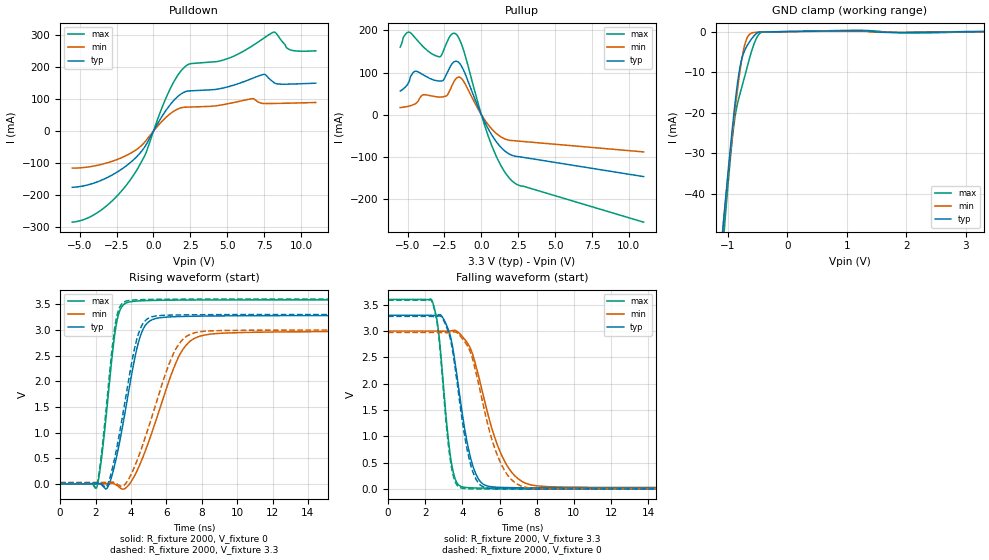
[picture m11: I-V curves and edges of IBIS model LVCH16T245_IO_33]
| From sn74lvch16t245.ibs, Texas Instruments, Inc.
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[Model]   LVCH16T245_IO_33
Model_type  I/O
Vinl=0.8
Vinh=2.0
Enable   Active-Low
Vref =   0
Rref =   2000
Cref =   15p
Vmeas =   1.5
| variable   typ   min   max
C_comp   6.04pF   5.05pF   7.40pF
| C_pullup   14.21pF   6.31pF   25.41pF
| C_pulldown   9.42pF   6.50pF   14.94pF
| C_tri-state   6.04pF   5.05pF   7.40pF
[Temperature Range]   40   100   -40
| Ambient temperature   25   85   -40
[Voltage range]   3.3   3   3.6
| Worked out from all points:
|   slope of the pulldown table from 0 to 0.495 V, typ, clamps not added: 12.4 ohm
|   slope of the pullup table from 0 to 0.495 V, typ, clamps not added: 14 ohm
|   GND clamp passes 1 mA (typ) near -0.56 V on its own axis
|   rising waveform, R_fixture 2000, V_fixture 0: 20-80 % time 1.06ns typ, 1.81ns min, 655ps max; typ from 0 V to 3.28 V
|   falling waveform, R_fixture 2000, V_fixture 3.3: 20-80 % time 887ps typ, 1.47ns min, 565ps max; typ from 3.3 V to 0.019 V
|   rising waveform, R_fixture 2000, V_fixture 3.3: 20-80 % time 1.03ns typ, 1.71ns min, 639ps max; typ from 0.019 V to 3.3 V
|   falling waveform, R_fixture 2000, V_fixture 0: 20-80 % time 841ps typ, 1.32ns min, 547ps max; typ from 3.28 V to 0 V
[GND Clamp]
| LVCH16T245_IO_33
|   Voltage   I(typ)   I(min)   I(max)
-5.5V     -898.4mA   -832.8mA   -1.017A
-1.095V   -50.42mA   -50.2mA    -55.28mA
-1.065V   -45.5mA    -45.64mA   -49.74mA
-1.04V    -41.45mA   -41.9mA    -45.21mA
-970mV    -30.49mA   -31.69mA   -33.19mA
-905mV    -21.04mA   -22.72mA   -23.79mA
-815mV    -10.36mA   -11.66mA   -16.39mA
-725mV    -4.895mA   -3.736mA   -11.48mA
-625mV    -2.267mA   -545.8uA   -5.994mA
-515mV    -439uA     -162.2uA   -1.527mA
-420mV    -95.51uA   -88.06uA   -143.5uA
3.3V      35.84pA    398.7nA    -4.252uA
[Pulldown]
| LVCH16T245_IO_33
|   Voltage   I(typ)   I(min)   I(max)
-5.5V     -176.2mA   -116.1mA   -285.6mA
-3.565V   -154.8mA   -104.8mA   -248.3mA
-1.62V    -100.7mA   -71.19mA   -156.1mA
-535mV    -45.52mA   -31.12mA   -71.38mA
1.155V    84.06mA    55.16mA    134.7mA
2.23V     124.7mA    75.07mA    205.2mA
5.1V      139.6mA    86.34mA    228.5mA
6.75V     166.1mA    101.8mA    268.8mA
7.495V    178.1mA    86.65mA    292mA
8.17V     152.3mA    86.77mA    310.5mA
9.2V      147.4mA    87.68mA    256mA
11V       150.3mA    89.74mA    251.8mA
[Pullup]
| LVCH16T245_IO_33
|   Voltage   I(typ)   I(min)   I(max)
-5.5V     56.18mA    16.98mA    160.3mA
-4.89V    79.66mA    20.64mA    195.7mA
-4.445V   103.3mA    26.89mA    180.5mA
-3.945V   94.62mA    47.4mA     161.1mA
-2.805V   79.84mA    41.85mA    137.4mA
-2.095V   114.9mA    61.02mA    187.6mA
-1.66V    126.5mA    87.57mA    189.1mA
-1.24V    108mA      81.18mA    156.3mA
695mV     -47.39mA   -33.41mA   -72.26mA
1.475V    -82.35mA   -55.39mA   -129.6mA
2.255V    -98mA      -61.58mA   -161.7mA
11V       -146.5mA   -88.02mA   -254.5mA
[Ramp]
| LVCH16T245_IO_33
| variable   typ   min   max
dV/dt_r   2.03/1.10E-09   1.85/1.88E-09   2.20/6.72E-10
dV/dt_f   1.97/8.89E-10   1.79/1.47E-09   2.16/5.70E-10
R_load = 2000
[Rising Waveform]
| LVCH16T245_IO_33
R_fixture =   2000
C_fixture =   0
L_fixture =   0
V_fixture =   0
V_fixture_min = 0
V_fixture_max = 0
|   Time   V(typ)   V(min)   V(max)
0s        381.8pV    6.463nV    1.925nV
2.075ns   863.6uV    142.5nV    -63.59mV
2.66ns    -78.85mV   298.8uV    1.528V
3.15ns    467.3mV    -17.38mV   3.059V
3.825ns   1.706V     -42.29mV   3.535V
4.395ns   2.719V     292.4mV    3.562V
4.9ns     3.124V     723.5mV    3.571V
6.69ns    3.259V     2.471V     3.58V
7.95ns    3.268V     2.882V     3.582V
34.99ns   3.279V     2.973V     3.584V
[Falling Waveform]
| LVCH16T245_IO_33
R_fixture =   2000
C_fixture =   0
L_fixture =   0
V_fixture =   3.3
V_fixture_min = 3
V_fixture_max = 3.6
|   Time   V(typ)   V(min)   V(max)
0s        3.3V       3V         3.6V
2.385ns   3.298V     3V         3.561V
2.72ns    3.309V     2.999V     2.983V
3.4ns     2.831V     3.004V     521.5mV
3.99ns    1.443V     2.899V     43.98mV
4.48ns    541.7mV    2.629V     25.31mV
4.975ns   139.7mV    1.998V     20.79mV
6.19ns    32.28mV    587mV      17.74mV
7.615ns   25.37mV    87.63mV    15.82mV
34.99ns   19.21mV    26.17mV    13.11mV
[Rising Waveform]
| LVCH16T245_IO_33
R_fixture =   2000
C_fixture =   0
L_fixture =   0
V_fixture =   3.3
V_fixture_min = 3
V_fixture_max = 3.6
|   Time   V(typ)   V(min)   V(max)
0s        19.15mV    25.82mV    13.1mV
2.065ns   19.8mV     25.82mV    -39.02mV
2.61ns    -56.69mV   25.69mV    1.497V
3.1ns     532.9mV    18.42mV    3.076V
3.75ns    1.78V      27.17mV    3.563V
4.295ns   2.771V     409.7mV    3.585V
4.77ns    3.165V     865.7mV    3.591V
6.41ns    3.289V     2.543V     3.597V
7.58ns    3.294V     2.941V     3.599V
34.99ns   3.3V       3V         3.6V
[Falling Waveform]
| LVCH16T245_IO_33
R_fixture =   2000
C_fixture =   0
L_fixture =   0
V_fixture =   0
V_fixture_min = 0
V_fixture_max = 0
|   Time   V(typ)   V(min)   V(max)
0s        3.279V     2.974V     3.585V
2.385ns   3.277V     2.974V     3.544V
2.715ns   3.288V     2.974V     2.953V
3.37ns    2.819V     2.975V     504.8mV
3.92ns    1.478V     2.892V     24.39mV
4.395ns   530.9mV    2.629V     7.08mV
4.875ns   111.4mV    1.994V     3.987mV
6.005ns   5.776mV    539.6mV    2.835mV
7.325ns   2.273mV    41.1mV     1.811mV
34.99ns   59.67uV    218.5uV    7.525uV
